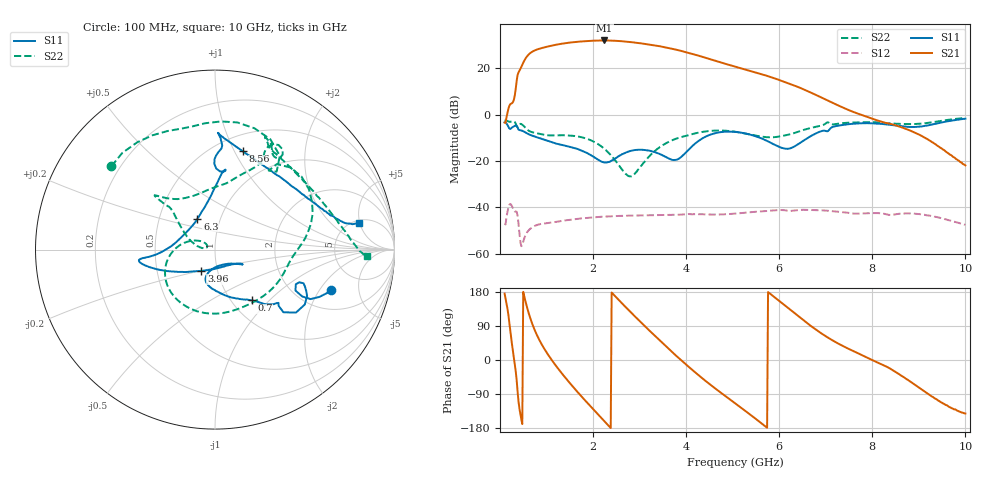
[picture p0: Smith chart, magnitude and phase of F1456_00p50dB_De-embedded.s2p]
! Integrated Device Technology
! Corporate Headquarters
! 6024 Silver Creek Valley Road
! San Jose, CA 95138  USA
! Phone:  1-408-284-8200
! Toll Free:  1-800-223-1366
! Webpage:  http://www.idt.com/
! Timing and RF Division
! 515 Groton Road, Suite 102
! Westford, MA 01886-6024
! Device:  F1456
! Description: 6-bit 0.5 dB Transmit Variable Gain Amplifier
! Frequency:  2100.0 -  2950.00 MHz
! Package:  6x6 mm Thin QFN Plastic Package: 28 pin
! State:  1
! Atten State:  0.5 dB
! Voltage:  +5.00 Volts
! Current:  212.985 mA
! Data:  The device was measured on a the F1455 evaluation board which has
!  individual transmission lines to the RF pins.  Data was collected
!  using a calibrated network analyzer.  The evaluation board was
!  de-embedded using a TRL calibration technique.
!  The reference plane is the edge of the package pin.
!  Pin  1 = CSb
!  Pin  2 = DATA
!  Pin  3 = CLK
!  Pin  4 = RSET
!  Pin  5 = GND
!  Pin  6 = RFIN  = Port 1
!  Pin  7 = GND
!  Pin  8 = NC
!  Pin  9 = NC
!  Pin 10 = NC
!  Pin 11 = NC
!  Pin 12 = NC
!  Pin 13 = NC
!  Pin 14 = /STBY
!  Pin 15 = GND
!  Pin 16 = RFOUT  = Port 2
!  Pin 17 = GND
!  Pin 18 = NC
!  Pin 19 = NC
!  Pin 20 = NC
!  Pin 21 = GND
!  Pin 22 = NC
!  Pin 23 = GND
!  Pin 24 = NC
!  Pin 25 = NC
!  Pin 26 = NC
!  Pin 27 = GND
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# GHz S dB R 50
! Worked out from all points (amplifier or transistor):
!   496 points, 100 MHz to 10 GHz, reference 50 ohm
!   highest |S21| = 32.0 dB at 2.24 GHz (marker M1)
!   |S21| within 3 dB of that: 950.9 MHz to 3.562 GHz (2.611 GHz wide, 116 % of centre)
!   unconditionally stable (mu >= 1): start of sweep to end of sweep
!   at 1.74 GHz: K = 2.18, MAG = 32.0 dB, |S12| = -44.9 dB
!   at 5.06 GHz: K = 4.47, MAG = 22.2 dB, |S12| = -42.7 dB
!   at 10 GHz: K = 144.32, MAG = -11.8 dB, |S12| = -47.5 dB
!   S11 on the Smith chart (normalised r, x): 100 MHz: 3.04, -2.56; 700 MHz: 1.23, -0.79; 3.96 GHz: 0.84, -0.20; 6.3 GHz: 0.78, +0.28; 8.56 GHz: 0.67, +1.08; 10 GHz: 5.38, +4.79
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0.1  -3.29 -19.1  -3.45 175.3  -47.18 40.8  -2.60 141.1
0.34  -4.64 -31.5  11.27 -30.7  -41.86 -142.4  -3.94 55.4
0.42  -6.71 -40.0  18.94 -129.5  -51.54 146.6  -4.13 47.3
0.56  -7.90 -48.3  24.52 149.1  -51.61 -175.5  -5.96 6.7
0.7  -9.18 -54.2  27.18 93.4  -48.55 145.8  -7.66 -12.9
0.94  -10.79 -68.9  28.91 32.2  -47.02 97.2  -8.73 -49.9
1.18  -12.39 -84.5  30.01 -11.4  -46.39 69.8  -8.97 -83.3
1.5  -13.93 -101.2  31.04 -60.8  -45.41 44.3  -9.05 -122.6
1.76  -15.61 -108.5  31.55 -97.3  -44.80 27.4  -9.82 -148.2
2.24  -20.67 -77.7  31.96 -161.1  -44.01 -0.1  -14.72 169.6
2.52  -18.41 -40.3  31.77 162.5  -43.77 -14.9  -20.90 149.0
2.84  -15.57 -29.4  31.19 122.4  -43.60 -30.6  -26.49 166.2
3.1  -15.26 -28.1  30.52 90.9  -43.49 -42.7  -20.55 169.3
3.4  -16.72 -32.6  29.59 55.4  -43.37 -56.2  -14.59 152.3
3.96  -17.03 -122.6  27.09 -8.0  -43.07 -79.8  -9.35 137.0
4.42  -9.52 -160.6  24.47 -55.5  -43.08 -101.4  -7.28 138.4
5.06  -7.48 -172.7  20.65 -114.9  -42.72 -125.8  -7.43 136.0
6.3  -14.05 119.7  12.69 126.6  -41.49 165.3  -8.12 77.1
6.7  -9.06 89.6  9.29 88.0  -41.15 138.7  -5.69 63.7
8.36  -4.37 82.2  -3.90 -21.0  -43.30 66.5  -3.79 62.3
8.56  -4.89 74.2  -5.03 -36.2  -42.88 62.5  -3.99 57.3
10  -1.79 10.7  -21.95 -141.3  -47.53 -16.9  -1.46 -2.5
